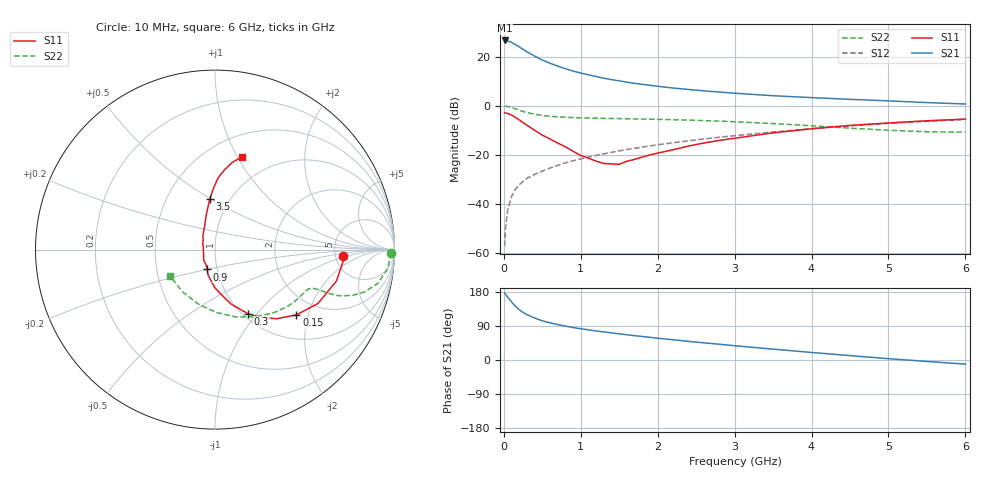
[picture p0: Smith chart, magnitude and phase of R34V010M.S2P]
! SIEMENS Small Signal Semiconductors
! BFR181
! Si NPN RF Bipolar Junction Transistor in SOT23
! VCE = 4 V  IC = 10 mA
! Common Emitter S-Parameters:  May  1996
# GHz  S  MA  R  50
!  f  S11  S21  S12  S22
! GHz  MAG  ANG  MAG  ANG  MAG  ANG  MAG  ANG
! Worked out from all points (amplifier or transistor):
!   36 points, 10 MHz to 6 GHz, reference 50 ohm
!   highest |S21| = 26.5 dB at 10 MHz (marker M1)
!   |S21| within 3 dB of that: start of sweep to 219.6 MHz
!   unconditionally stable (mu >= 1): 816.6 MHz to 2.661 GHz
!   at 250 MHz: K = 0.61, MSG = 26.8 dB, |S12| = -30.8 dB
!   at 1.4 GHz: K = 1.06, MAG = 13.3 dB, |S12| = -18.9 dB
!   at 6 GHz: K = 0.85, MSG = 3.1 dB, |S12| = -5.6 dB
!   S11 on the Smith chart (normalised r, x): 10 MHz: 5.93, -0.85; 150 MHz: 1.54, -1.69; 300 MHz: 1.06, -0.90; 900 MHz: 0.90, -0.20; 3.5 GHz: 0.81, +0.49; 6 GHz: 0.72, +1.04
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0.01  0.7165 -2.8  21.26 176.8  0.0014 103.9  0.9831 -1.1
0.02  0.7158 -5.6  20.97 173.9  0.0031 85.8  0.9765 -2.5
0.05  0.6989 -14.5  20.75 166.0  0.0077 84.1  0.9681 -6.3
0.1  0.6477 -27.6  19.43 153.4  0.0143 78.6  0.9253 -11.8
0.15  0.5816 -38.7  17.52 141.8  0.0202 72.5  0.8665 -15.8
0.2  0.5153 -48.4  15.75 133.0  0.0247 71.0  0.8127 -18.2
0.25  0.4544 -56.0  14.01 125.6  0.029 69.3  0.7644 -19.7
0.3  0.4029 -62.7  12.5 119.8  0.0335 68.7  0.7278 -20.6
0.4  0.3175 -73.4  10.23 110.9  0.0404 68.1  0.6739 -21.1
0.5  0.2529 -82.1  8.504 103.4  0.047 69.0  0.6356 -21.1
0.6  0.2115 -90.3  7.322 98.1  0.0542 69.2  0.6118 -21.2
0.7  0.174 -97.4  6.404 93.5  0.0615 69.5  0.5962 -21.4
0.9  0.119 -111.3  5.077 85.6  0.0761 69.8  0.5757 -22.0
1.1  0.0862 -137.4  4.259 79.6  0.0905 70.1  0.5633 -23.2
1.3  0.0671 -161.9  3.641 74.2  0.1057 69.8  0.5539 -24.8
1.6  0.0747 155.6  3.016 66.5  0.1289 68.8  0.5444 -28.0
2.2  0.1275 119.0  2.294 53.4  0.1774 65.6  0.5209 -35.7
2.6  0.1749 107.6  2.009 45.3  0.2115 62.6  0.4983 -41.7
3.5  0.2815 96.0  1.6 28.6  0.2927 54.9  0.4349 -59.3
4.5  0.3987 87.6  1.351 11.6  0.39 44.0  0.3504 -88.7
5.5  0.4952 78.8  1.161 -3.9  0.4844 31.2  0.2964 -128.1
6  0.536 74.0  1.086 -10.9  0.5277 24.2  0.291 -150.1
